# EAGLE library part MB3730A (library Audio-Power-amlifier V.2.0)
FUJITSU - 1,4 BTL AUDIO POWER AMPLIEFIER
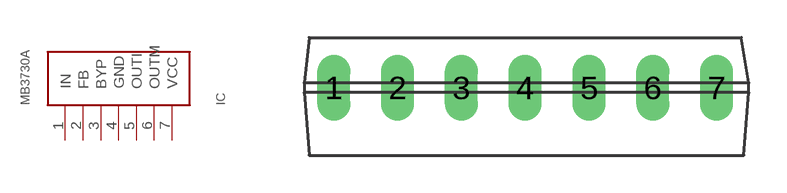
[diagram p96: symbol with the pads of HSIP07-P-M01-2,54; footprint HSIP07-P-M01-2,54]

Designator prefix IC

## MB3730ASIP7  [HSIP07-P-M01-2,54]
1  IN  in
2  FB
3  BYP
4  GND  pwr
5  OUTI  out
6  OUTM  out
7  VCC  pwr

## Footprint HSIP07-P-M01-2,54 (pad centres in mm)
drill 0.8 long: 1 -7.62,0; 2 -5.08,0; 3 -2.54,0; 4 0,0; 5 2.54,0; 6 5.08,0; 7 7.62,0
